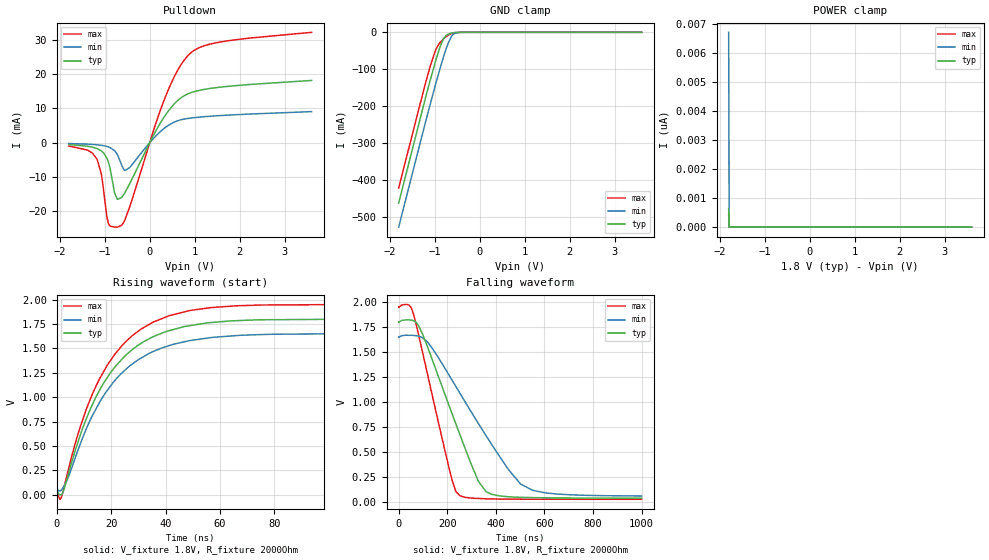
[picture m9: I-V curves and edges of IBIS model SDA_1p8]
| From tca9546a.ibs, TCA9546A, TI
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|   Model
[Model]   SDA_1p8
Model_type   I/O_open_drain
Polarity   Non-Inverting
Enable   Active-Low
Vinl = 0.54
Vinh = 1.26
Vmeas = 0.9
Vref = 1.8
Cref = 1pF
Rref = 2000
|   typ   min   max
C_comp   3.666pF   3.611pF   3.839pF
[Voltage Range]   1.8   1.65   1.95
[Temperature Range]   27   125   -40
[Pullup Reference]   1.8   1.65   1.95
[Pulldown Reference]   -0   -0   -0
[Power Clamp Reference]   1.8   1.65   1.95
[GND Clamp Reference]   -0   -0   -0
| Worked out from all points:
|   slope of the pulldown table from 0 to 0.27 V, typ, clamps not added: 41.8 ohm
|   GND clamp passes 1 mA (typ) near -0.58 V on its own axis
|   falling waveform, V_fixture 1.8V, R_fixture 2000Ohm: 20-80 % time 162ns typ, 245ns min, 108ns max; typ from 1.8 V to 0.034 V
|   rising waveform, V_fixture 1.8V, R_fixture 2000Ohm: 20-80 % time 19.9ns typ, 20.6ns min, 19.5ns max; typ from 0.034 V to 1.8 V
[Pulldown]
|   Voltage   I(typ)   I(min)   I(max)
-1.8V     -559.3uA   -253uA     -973.1uA
-1.379V   -1.039mA   -424.7uA   -2.167mA
-1.174V   -1.711mA   -614.3uA   -4.774mA
-1.076V   -2.404mA   -768.8uA   -9.084mA
-919.8mV  -5.603mA   -1.238mA   -23.36mA
-779.4mV  -14.76mA   -2.357mA   -24.62mA
-628.2mV  -15.99mA   -6.339mA   -24.11mA
-450mV    -12.1mA    -7.326mA   -18.9mA
349.2mV   8.042mA    4.436mA    13.39mA
851.4mV   14.24mA    7.062mA    25.39mA
1.516V    16.09mA    7.853mA    29.2mA
3.595V    18.13mA    9.046mA    32.14mA
[GND Clamp]
|   Voltage   I(typ)   I(min)   I(max)
-1.8V     -462.4mA   -527.7mA   -421.6mA
-1.244V   -196.1mA   -261.8mA   -156mA
-1.093V   -126.8mA   -191.7mA   -89.3mA
-1.001V   -86.68mA   -150.1mA   -54.73mA
-946.8mV  -64.38mA   -126.2mA   -39.76mA
-882mV    -40.04mA   -98.29mA   -28.02mA
-795.6mV  -15.96mA   -63.07mA   -16.94mA
-703.8mV  -5.168mA   -30.46mA   -7.977mA
-628.2mV  -1.927mA   -11.24mA   -3.14mA
-558mV    -623.1uA   -2.801mA   -927.7uA
-363.6mV  -8.702uA   -29.31uA   -7.74uA
3.595V    0A         0A         0A
[POWER Clamp]
|   Voltage   I(typ)   I(min)   I(max)
-1.8V     629.4pA    6.714nA    447.8pA
-1.789V   0A         0A         0A
-1.784V   0A         0A         0A
3.595V    0A         0A         0A
[Ramp]
R_load = 2000
|   typ   min   max
dV/dt_r   1.05976/1.99378e-08   0.956666/2.05316e-08   1.15654/1.954e-08
dV/dt_f   1.05975/1.62203e-07   0.956624/2.45268e-07   1.15654/1.08431e-07
[Falling Waveform]
V_fixture = 1.8V
V_fixture_min = 1.65V
V_fixture_max = 1.95V
R_fixture = 2000Ohm
C_fixture = 0F
|   Time   V(typ)   V(min)   V(max)
0s        1.8V       1.65V      1.95V
56.63ns   1.817V     1.667V     1.915V
118.5ns   1.552V     1.6V       1.279V
218.9ns   887.1mV    1.221V     223.3mV
251.9ns   671.5mV    1.087V     59.52mV
327.6ns   204.6mV    784.8mV    31.27mV
360ns     98.67mV    659.6mV    27.64mV
502.4ns   42.58mV    174.2mV    23.82mV
651.7ns   36.14mV    75.5mV     23.13mV
1us       33.75mV    55.62mV    22.44mV
[Rising Waveform]
V_fixture = 1.8V
V_fixture_min = 1.65V
V_fixture_max = 1.95V
R_fixture = 2000Ohm
C_fixture = 0F
|   Time   V(typ)   V(min)   V(max)
0s        33.73mV    55.54mV    22.44mV
1.704ns   -797.2uV   47.13mV    -30.09mV
3.84ns    160mV      147.9mV    199.1mV
8.547ns   596.2mV    507.9mV    681.7mV
13.99ns   972.9mV    853.8mV    1.085V
24.03ns   1.39V      1.25V      1.529V
30.92ns   1.55V      1.399V     1.696V
41.52ns   1.684V     1.53V      1.838V
65.83ns   1.784V     1.631V     1.937V
1us       1.8V       1.65V      1.95V
